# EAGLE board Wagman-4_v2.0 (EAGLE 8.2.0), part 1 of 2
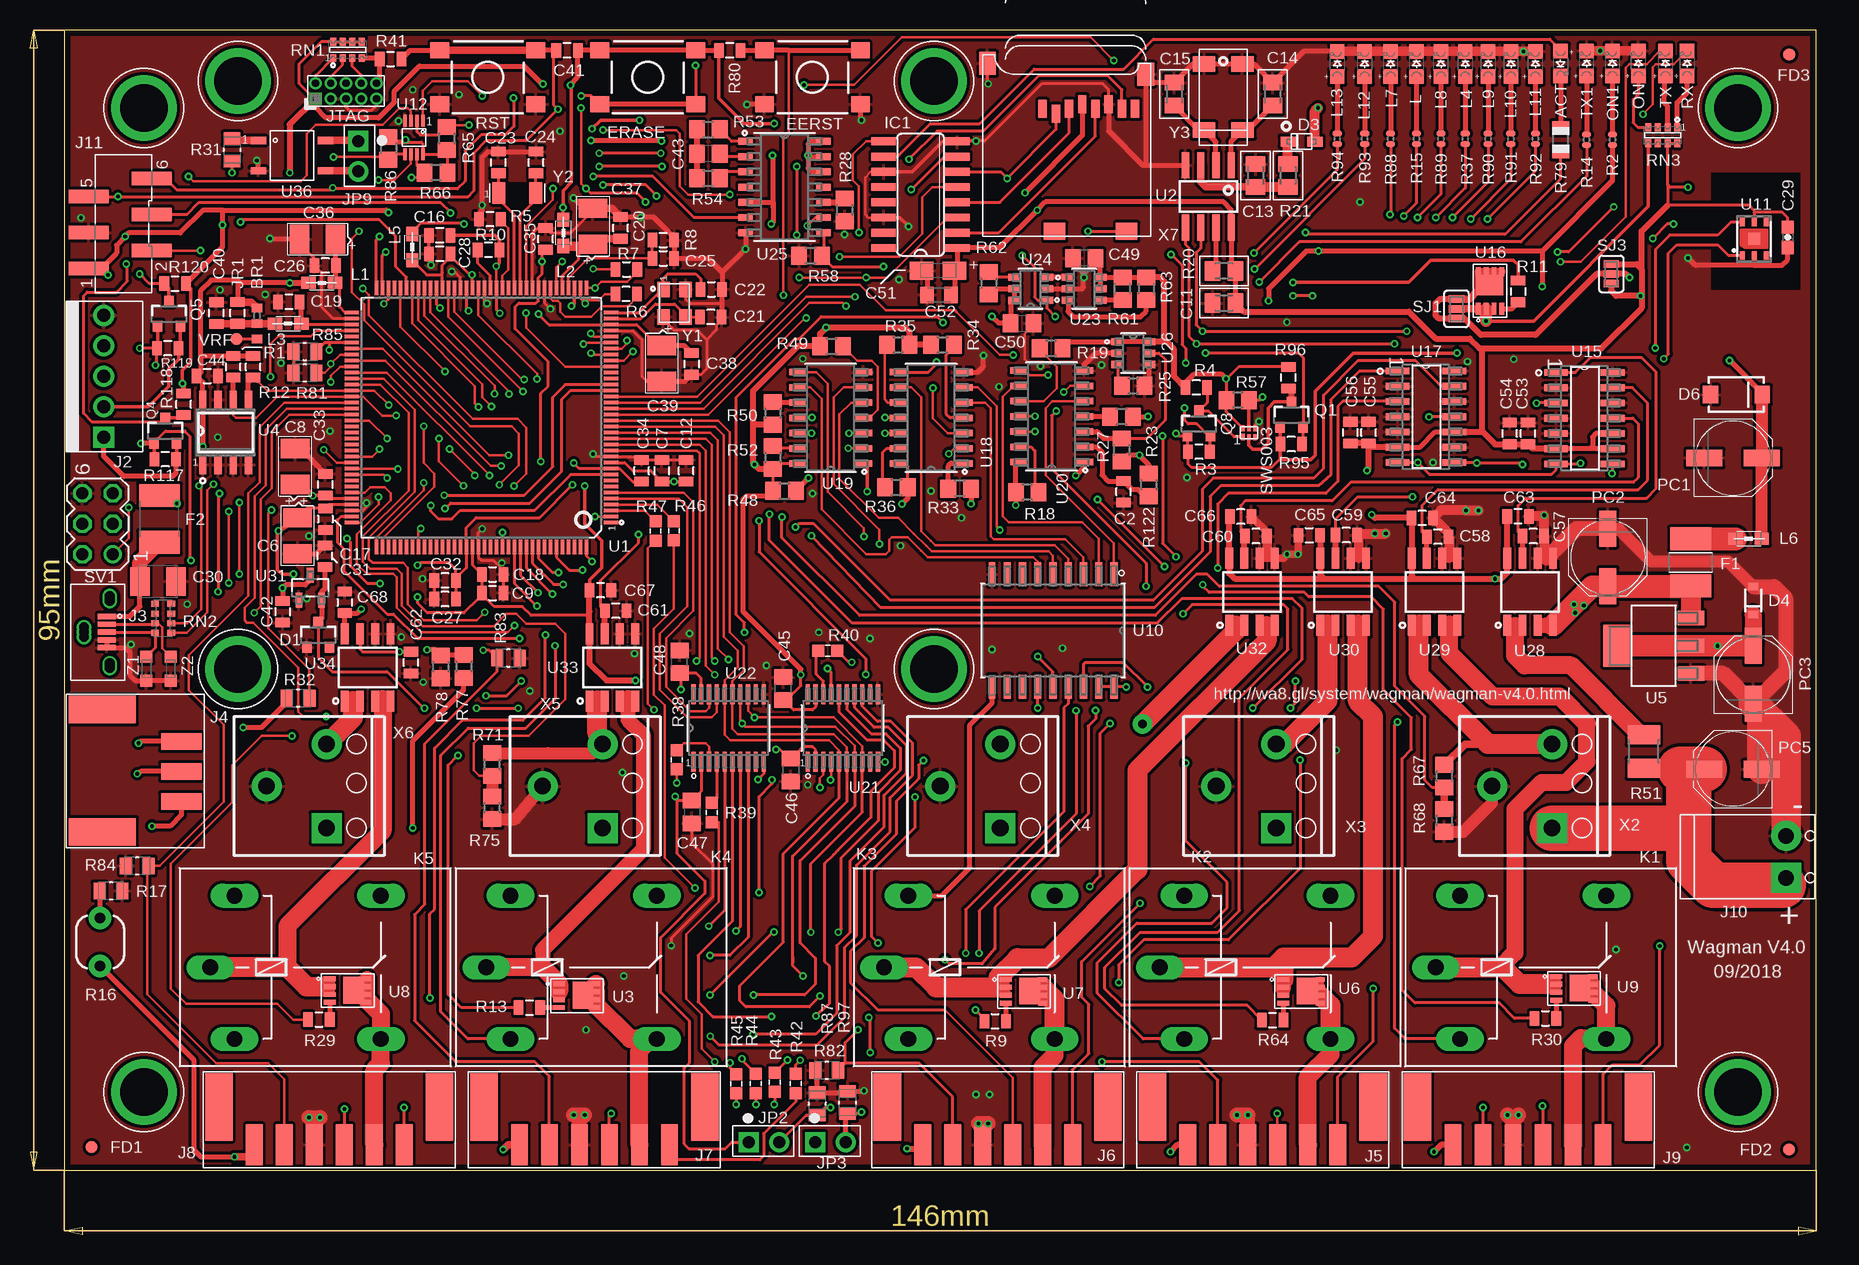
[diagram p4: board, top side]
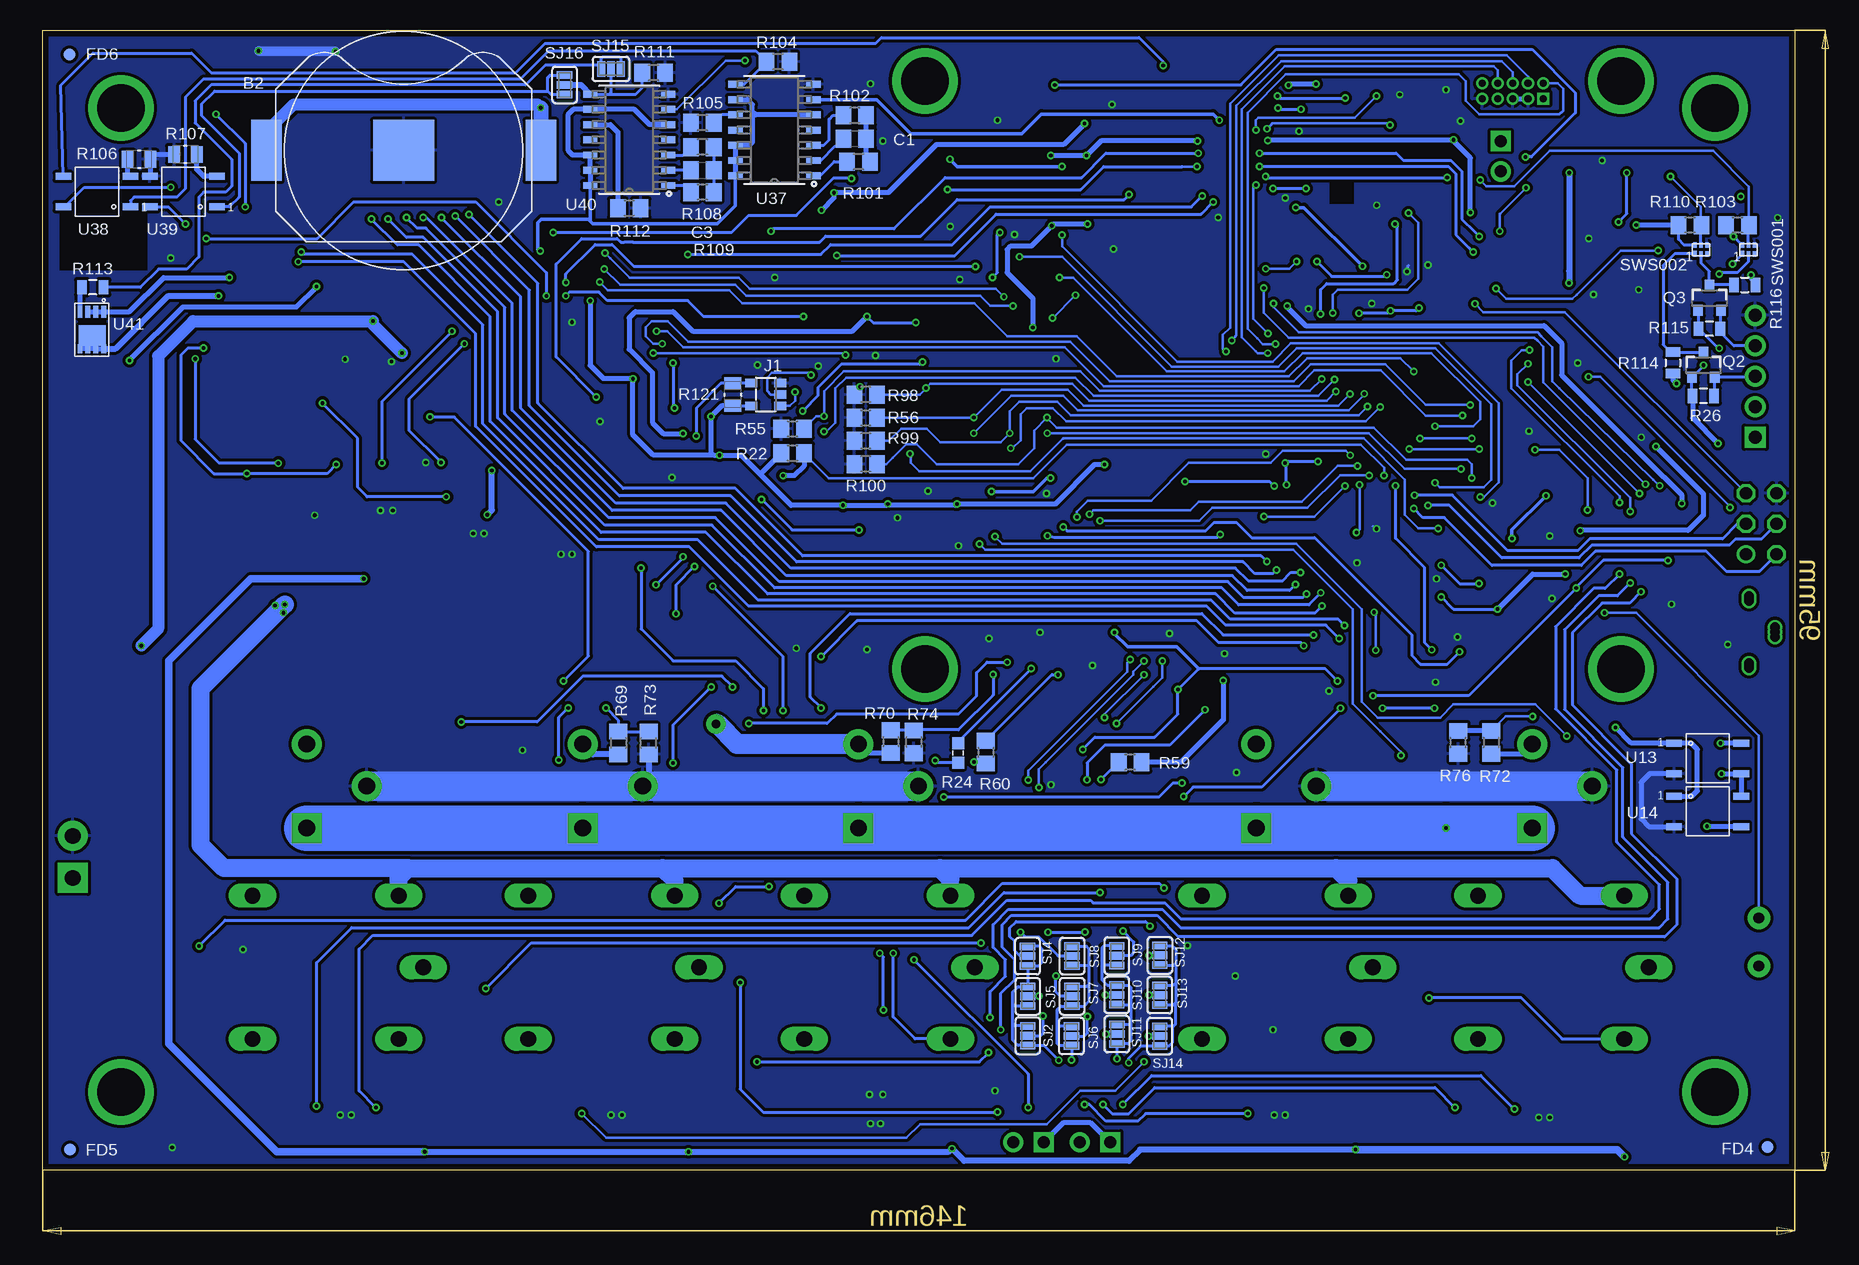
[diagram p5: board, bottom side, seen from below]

Size 148.84 x 100.38 mm. Coordinates in mm from the lower left corner, seen from the top.
Outline: 2.84,5.38 148.84,5.38 148.84,100.38 2.84,100.38 2.84,5.38
Copper layers (1*16): Top 0.035mm / dielectric 1.5mm / Bottom 0.035mm
Design rules "default *": minimum track width 0.2mm, minimum drill 12mil, track to track 10mil, track to pad 10mil, pad to pad 10mil, via to via 10mil, smd to smd 0mil, copper to edge 20mil, drill to drill 10mil, minimum pad ring 5mil, minimum via ring 5mil, stop-mask expansion 2.5mil, vias tented up to drill 0mil, thermal gap 10mil
tRestrict: area 140.1,78.7 to 147.5,88.5
bRestrict: area 140.1,80.4 to 147.4,85.3

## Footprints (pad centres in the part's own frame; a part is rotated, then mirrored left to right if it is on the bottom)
CHIPLED_0805 = smd 1.2 x 1.2: A 0,-1.05; C 0,1.05
BAT-HLD-002-SMT = smd 5.08 x 5.08: NEG 0,0 | smd 2.54 x 5.08: POS1 -11.43,0; POS2 11.43,0
J0402 = smd 0.7 x 0.9: 1 -0.65,0; 2 0.65,0; 3 1.95,0
C0805 = smd 1.3 x 1.5: 1 -0.95,0; 2 0.95,0
0805 = smd 0.8 x 1.2: 1 -0.9,0; 2 0.9,0
SMC_B = smd 1.6 x 2.4: + -1.5,0; - 1.5,0
M0805 = smd 1.3 x 1.6: 1 -0.95,0; 2 0.95,0
0603-CAP = smd 1.1 x 1: 1 -0.85,0; 2 0.85,0
A/3216-18R = smd 1.95 x 1.5: + 1.375,0; - -1.375,0
C0805K = smd 1.1 x 1.4: 1 -1,0; 2 1,0
SOT23-3 = smd 0.8 x 0.9: 1 -0.95,-1; 2 0.95,-1; 3 0,1.1
SOD-323F = smd 1.27 x 0.813: A -1.118,0; K 1.118,0
SOD-323 = smd 0.63 x 0.83: A 1.15,0; C -1.15,0
SMA-DIODE = smd 1.27 x 1.47: A -2.15,0; C 2.15,0
TACT_SPST_SMD_6X6 = smd 1.55 x 1.3: 1 -4,2.25; 2 4,2.25; 3 4,-2.25; 4 -4,-2.25
L1812 = smd 1.9 x 3.4: 1 -1.95,0; 2 1.95,0
FD-1MM = smd 1 x 1: 1 0,0
SO16 = smd 0.66 x 2.032: 1 -4.445,-3.073; 2 -3.175,-3.073; 3 -1.905,-3.073; 4 -0.635,-3.073; 5 0.635,-3.073; 6 1.905,-3.073; 7 3.175,-3.073; 8 4.445,-3.073; 9 4.445,3.073; 10 3.175,3.073; 11 1.905,3.073; 12 0.635,3.073; 13 -0.635,3.073; 14 -1.905,3.073; 15 -3.175,3.073; 16 -4.445,3.073
TSOP-5 = smd 0.7 x 1: 1 -0.95,-1.2; 2 0,-1.2; 3 0.95,-1.2; 4 0.95,1.2; 5 -0.95,1.2
01X05_P2.54_RELIMATE = drill 1.1 pad 1.778 square: 1 -5.08,0 | drill 1.1 pad 1.778: 2 -2.54,0; 3 0,0; 4 2.54,0; 5 5.08,0
1051330011_MINIUSB_VERTICAL = smd 0.45 x 1.5: 1 -1.3,0; 2 -0.65,0; 3 0,0; 4 0.65,0; 5 1.3,0 | drill 0.8: 6 -2.6,0.25; 7 3,0.25; 8 -3,0.25; 9 -2.8,0.25; 10 2.6,0.25; 11 2.8,0.25; 12 0.4,-1.9; 13 -0.4,-1.9; 14 0,-1.9
3PIN-PTSM-RA-2.5MM = smd 1.4 x 3.4: 1 -2.44,0; 2 0.06,0; 3 2.56,0 | smd 2.3 x 5.6: M1 -5.1,-6.6; M2 5.1,-6.6
6PIN-PTSM-2.5MM = smd 1.4 x 3.4: 1 -6.25,0; 2 -3.75,0; 3 -1.25,0; 4 1.25,0; 5 3.75,0; 6 6.25,0 | smd 2.3 x 5.6: M1 -9.2,-3.15; M2 9.2,-3.15
TB2-3.5MM = drill 1.3 pad 2.5 square: P$1 -1.75,0 | drill 1.3 pad 2.5: P$2 1.75,0
1X6-STRAIGHT-ALT = smd 1.1 x 3.3: 1 3.75,-2.9; 2 2.25,2.35; 3 0.75,-2.9; 4 -0.75,2.35; 5 -2.25,-2.9; 6 -3.75,2.35
CONN_2PIN_P2.54MM = drill 1 pad 1.676 square: 1 0,0 | drill 1 pad 1.676: 2 2.54,0
PINHEAD_2X05_127 = drill 0.6 pad 1.016 square: 1 -0.635,2.54 | drill 0.6 pad 1.016: 2 0.635,2.54; 3 -0.635,1.27; 4 0.635,1.27; 5 -0.635,0; 6 0.635,0; 7 -0.635,-1.27; 8 0.635,-1.27; 9 -0.635,-2.54; 10 0.635,-2.54
G5LE = drill 1.321 long: 1 -7.493,-5.969; 2 -7.493,5.969; O 4.699,5.969; P -9.525,0; S 4.699,-5.969
0805' = smd 1.2 x 1: 1 -1.1,0; 2 1.1,0
MH3.964 = drill 3.962 pad 5.461: 1 0,0
PANASONIC_D = smd 3 x 1.4: + 2.4,0; - -2.4,0
R0402 = smd 0.508 x 0.762: 1 -0.445,0; 2 0.445,0
PHOTOCELL-KIT = drill 0.9 pad 1.88: 1 -2,0; 2 2,0
RESC2013X65N = smd 1.016 x 1.397: 1 -0.94,0; 2 0.94,0
R0805 = smd 1.3 x 1.5: 1 -0.95,0; 2 0.95,0
PTC-0603 = smd 1 x 1: 1 -0.8,0; 2 0.8,0
R1210 = smd 1.6 x 2.7: 1 -1.4,0; 2 1.4,0
R0805' = smd 1.1 x 1.4: 1 -1,0; 2 1,0
CAT16 = smd 0.5 x 0.65: 1 -1.2,-0.675; 2 -0.4,-0.675; 3 0.4,-0.675; 4 1.2,-0.675; 5 1.2,0.675; 6 0.4,0.675; 7 -0.4,0.675; 8 -1.2,0.675
CAY16 = smd 0.5 x 0.65: 1 -1.2,-0.675; 2 -0.4,-0.675; 3 0.4,-0.675; 4 1.2,-0.675; 5 1.2,0.675; 6 0.4,0.675; 7 -0.4,0.675; 8 -1.2,0.675
SJ_3_PASTE1&2&3 = smd 0.635 x 1.27: 1 -0.813,0; 2 0,0; 3 0.813,0
MA03-2 = drill 1.016: 1 -2.54,-1.27 | drill 1.016 octagon: 2 -2.54,1.27; 3 0,-1.27; 4 0,1.27; 5 2.54,-1.27; 6 2.54,1.27
CAT872 = smd 0.3 x 0.53: 1 -0.5,-0.355 | smd 0.3 x 0.49: 2 0,-0.375; 3 0.5,-0.375; 4 0.5,0.375; 5 0,0.375; 6 -0.5,0.375
LQFP144 = smd 0.3 x 1.2: 1 -8.75,-10.8; 2 -8.25,-10.8; 3 -7.75,-10.8; 4 -7.25,-10.8; 5 -6.75,-10.8; 6 -6.25,-10.8; 7 -5.75,-10.8; 8 -5.25,-10.8; 9 -4.75,-10.8; 10 -4.25,-10.8; 11 -3.75,-10.8; 12 -3.25,-10.8; 13 -2.75,-10.8; 14 -2.25,-10.8; 15 -1.75,-10.8; 16 -1.25,-10.8; 17 -0.75,-10.8; 18 -0.25,-10.8; 19 0.25,-10.8; 20 0.75,-10.8; 21 1.25,-10.8; 22 1.75,-10.8; 23 2.25,-10.8; 24 2.75,-10.8; 25 3.25,-10.8; 26 3.75,-10.8; 27 4.25,-10.8; 28 4.75,-10.8; 29 5.25,-10.8; 30 5.75,-10.8; 31 6.25,-10.8; 32 6.75,-10.8; 33 7.25,-10.8; 34 7.75,-10.8; 35 8.25,-10.8; 36 8.75,-10.8; 73 8.75,10.8; 74 8.25,10.8; 75 7.75,10.8; 76 7.25,10.8; 77 6.75,10.8; 78 6.25,10.8; 79 5.75,10.8; 80 5.25,10.8; 81 4.75,10.8; 82 4.25,10.8; 83 3.75,10.8; 84 3.25,10.8; 85 2.75,10.8; 86 2.25,10.8; 87 1.75,10.8; 88 1.25,10.8; 89 0.75,10.8; 90 0.25,10.8; 91 -0.25,10.8; 92 -0.75,10.8; 93 -1.25,10.8; 94 -1.75,10.8; 95 -2.25,10.8; 96 -2.75,10.8; 97 -3.25,10.8; 98 -3.75,10.8; 99 -4.25,10.8; 100 -4.75,10.8; 101 -5.25,10.8; 102 -5.75,10.8; 103 -6.25,10.8; 104 -6.75,10.8; 105 -7.25,10.8; 106 -7.75,10.8; 107 -8.25,10.8; 108 -8.75,10.8 | smd 1.2 x 0.3: 37 10.8,-8.75; 38 10.8,-8.25; 39 10.8,-7.75; 40 10.8,-7.25; 41 10.8,-6.75; 42 10.8,-6.25; 43 10.8,-5.75; 44 10.8,-5.25; 45 10.8,-4.75; 46 10.8,-4.25; 47 10.8,-3.75; 48 10.8,-3.25; 49 10.8,-2.75; 50 10.8,-2.25; 51 10.8,-1.75; 52 10.8,-1.25; 53 10.8,-0.75; 54 10.8,-0.25; 55 10.8,0.25; 56 10.8,0.75; 57 10.8,1.25; 58 10.8,1.75; 59 10.8,2.25; 60 10.8,2.75; 61 10.8,3.25; 62 10.8,3.75; 63 10.8,4.25; 64 10.8,4.75; 65 10.8,5.25; 66 10.8,5.75; 67 10.8,6.25; 68 10.8,6.75; 69 10.8,7.25; 70 10.8,7.75; 71 10.8,8.25; 72 10.8,8.75; 109 -10.8,8.75; 110 -10.8,8.25; 111 -10.8,7.75; 112 -10.8,7.25; 113 -10.8,6.75; 114 -10.8,6.25; 115 -10.8,5.75; 116 -10.8,5.25; 117 -10.8,4.75; 118 -10.8,4.25; 119 -10.8,3.75; 120 -10.8,3.25; 121 -10.8,2.75; 122 -10.8,2.25; 123 -10.8,1.75; 124 -10.8,1.25; 125 -10.8,0.75; 126 -10.8,0.25; 127 -10.8,-0.25; 128 -10.8,-0.75; 129 -10.8,-1.25; 130 -10.8,-1.75; 131 -10.8,-2.25; 132 -10.8,-2.75; 133 -10.8,-3.25; 134 -10.8,-3.75; 135 -10.8,-4.25; 136 -10.8,-4.75; 137 -10.8,-5.25; 138 -10.8,-5.75; 139 -10.8,-6.25; 140 -10.8,-6.75; 141 -10.8,-7.25; 142 -10.8,-7.75; 143 -10.8,-8.25; 144 -10.8,-8.75
SO08 = smd 0.6 x 2.2: 1 -1.905,-2.6; 2 -0.635,-2.6; 3 0.635,-2.6; 4 1.905,-2.6; 5 1.905,2.6; 6 0.635,2.6; 7 -0.635,2.6; 8 -1.905,2.6
SIS413 = smd 0.99 x 0.405: 1 0,0; 2 0,-0.66; 3 0,-1.32; 4 0,-1.98 | smd 0.76 x 0.405: 5 3.075,-1.98; 6 3.075,-1.32; 7 3.075,-0.66; 8 3.075,0 | smd 1.725 x 2.235: PAD 1.992,-0.96
SOIC8 = smd 0.6 x 1.55: 1 -1.905,-2.7; 2 -0.635,-2.7; 3 0.635,-2.7; 4 1.905,-2.7; 5 1.905,2.7; 6 0.635,2.7; 7 -0.635,2.7; 8 -1.905,2.7
SOT230P700X180-4N = smd 2.2 x 1.2: 1 -3.1,2.311; 2 -3.1,0; 3 -3.1,-2.311 | smd 2.2 x 3.5: 4 3.1,0
DW18 = smd 2 x 0.6: 1 -4.7,5.08; 2 -4.7,3.81; 3 -4.7,2.54; 4 -4.7,1.27; 5 -4.7,0; 6 -4.7,-1.27; 7 -4.7,-2.54; 8 -4.7,-3.81; 11 4.7,-3.81; 12 4.7,-2.54; 13 4.7,-1.27; 14 4.7,0; 15 4.7,1.27; 16 4.7,2.54; 17 4.7,3.81; 18 4.7,5.08 | smd 1.95 x 0.55: 9 -4.7,-5.08; 10 4.7,-5.08
DD8-3X3MM = smd 0.4 x 0.7: 1 -1,-1.4; 2 0,-1.4; 3 1,-1.4; 4 1,1.4; 5 0,1.4; 6 -1,1.4 | smd 1 x 1: EXP 0,0
US-8 = smd 0.3 x 1: 1 -0.75,-1.4; 2 -0.25,-1.4; 3 0.25,-1.4; 4 0.75,-1.4; 5 0.75,1.4; 6 0.25,1.4; 7 -0.25,1.4; 8 -0.75,1.4
SOP-4 = smd 1.3 x 0.6: 1 0,0; 2 0,-2.54; 3 5.6,-2.54; 4 5.6,0
SOIC127P600X175-14N = smd 1.981 x 0.559: 1 -2.362,3.81; 2 -2.362,2.54; 3 -2.362,1.27; 4 -2.362,0; 5 -2.362,-1.27; 6 -2.362,-2.54; 7 -2.362,-3.81; 8 2.362,-3.81; 9 2.362,-2.54; 10 2.362,-1.27; 11 2.362,0; 12 2.362,1.27; 13 2.362,2.54; 14 2.362,3.81
D14 = smd 1.5 x 0.55: 1 -2.7,3.81; 2 -2.7,2.54; 3 -2.7,1.27; 4 -2.7,0; 5 -2.7,-1.27; 6 -2.7,-2.54; 7 -2.7,-3.81; 8 2.7,-3.81; 9 2.7,-2.54; 10 2.7,-1.27; 11 2.7,0; 12 2.7,1.27; 13 2.7,2.54; 14 2.7,3.81
PW20 = smd 1.676 x 0.356: 1 -2.819,2.925; 2 -2.819,2.275; 3 -2.819,1.625; 4 -2.819,0.975; 5 -2.819,0.325; 6 -2.819,-0.325; 7 -2.819,-0.975; 8 -2.819,-1.625; 9 -2.819,-2.275; 10 -2.819,-2.925; 11 2.819,-2.925; 12 2.819,-2.275; 13 2.819,-1.625; 14 2.819,-0.975; 15 2.819,-0.325; 16 2.819,0.325; 17 2.819,0.975; 18 2.819,1.625; 19 2.819,2.275; 20 2.819,2.925
DBV6 = smd 1.05 x 0.6: 1 -1.35,0.95; 2 -1.35,0; 3 -1.35,-0.95; 4 1.35,-0.95; 5 1.35,0; 6 1.35,0.95
SOIC14-3.9MM = smd 1.2 x 0.58: 1 -3.25,3.81; 2 -3.25,2.54; 3 -3.25,1.27; 4 -3.25,0; 5 -3.25,-1.27; 6 -3.25,-2.54; 7 -3.25,-3.81; 8 3.25,-3.81; 9 3.25,-2.54; 10 3.25,-1.27; 11 3.25,0; 12 3.25,1.27; 13 3.25,2.54; 14 3.25,3.81
DDC6 = smd 1.05 x 0.6: 1 -1.3,0.95; 2 -1.3,0; 3 -1.3,-0.95; 4 1.3,-0.95; 5 1.3,0; 6 1.3,0.95
SOIC-8 = smd 1.75 x 0.65: 1 -2.8,1.905; 2 -2.8,0.635; 3 -2.8,-0.635; 4 -2.8,-1.905; 5 2.8,-1.905; 6 2.8,-0.635; 7 2.8,0.635; 8 2.8,1.905
SOT95P237X112-3N = smd 0.559 x 1.27: 1 -0.94,-1.041; 2 0.94,-1.041; 3 0,1.041
1-2834019-3 = drill 1.4 pad 2.5 square: 1 -3.5,0 | drill 1.4 pad 2.5: 2 0,5; 3 3.5,0
MICROSD = smd 0.7 x 1.5: 1 9,-10.64; 2 7.9,-10.24; 3 6.8,-10.64; 4 5.7,-11.04; 5 4.6,-10.64; 6 3.5,-11.04; 7 2.4,-10.64; 8 1.3,-10.64 | smd 1.8 x 1.4: CD1 2,-0.44; CD2 8,-0.44 | smd 1.4 x 1.9: MT1 0.4,-13.54; MT2 13.6,-14.44
CRYSTAL-3.2-2.5 = smd 1.3 x 1.05: 1 -1.15,-0.925; 2 1.15,-0.925; 3 1.15,0.925; 4 -1.15,0.925
RESONATOR_EPSON_FC_145 = smd 1.1 x 1.8: P$1 -1.55,0; P$2 1.55,0
CRYSTAL-CITIZEN-CM2XXC = smd 1.3 x 1.9: P$1 -2.75,-1.6; P$2 2.75,-1.6; P$3 2.75,1.6; P$4 -2.75,1.6
CT/CN0603 = smd 1 x 1: 1 -1,0; 2 1,0

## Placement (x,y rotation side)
ACT  RED  [CHIPLED_0805]  127.55,97.58 180 top
B2  CR2016  [BAT-HLD-002-SMT]  118.77,90.34 180 bottom
BR1  NM  [J0402]  18.92,75.27 90 top
C1  10nF  [C0805]  81.17,91.33 0 bottom
C2  10uF  [0805]  91.13,61.89 90 top
C3  10nF  [C0805]  93.87,88.69 0 bottom
C6  10u  [SMC_B]  22.29,58.24 270 top
C7  100nF  [0805]  52.65,63.65 90 top
C8  10u  [SMC_B]  22.09,64.01 90 top
C9  100nF  [0805]  38.55,53.46 0 top
C11  100nF  [M0805]  99.49,77.62 180 top
C12  100nF  [0805]  54.68,63.65 90 top
C13  100pF  [M0805]  102.13,88.26 90 top
C14  10pF  [M0805]  103.55,95.04 90 top
C15  8.2pF  [M0805]  95.35,95.04 90 top
C16  100nF  [0805]  34.15,83.26 180 top
C17  100nF  [0805]  24.61,59.62 270 top
C18  100nF  [0805]  38.55,55.01 0 top
C19  100nF  [0805]  21.57,77.72 180 top
C20  100nF  [0805]  49.22,83.88 90 top
C21  22pF  [0805]  56.74,76.46 180 top
C22  22pF  [0805]  56.78,78.76 0 top
C23  22pF  [0805]  39.03,89.35 90 top
C24  22pF  [0805]  42.18,89.35 90 top
C25  22pF  [0805]  52.77,81.35 0 top
C26  100nF  [0805]  24.6,80.75 180 top
C27  100nF  [0805]  34.59,52.96 180 top
C28  100nF  [0805]  34.14,81.73 180 top
C29  100nF  [0603-CAP]  146.48,83.1 270 top
C30  10nF  [SMC_B]  10.66,54.43 0 top
C31  1uF  [0805]  24.57,56.54 90 top
C32  100nF  [0805]  34.59,54.51 180 top
C33  100nF  [0805]  24.61,62.5 90 top
C34  100nF  [0805]  50.97,63.65 90 top
C35  100nF  [0805]  42.97,82.97 90 top
C36  10u  [SMC_B]  23.96,82.94 180 top
C37  10u  [SMC_B]  46.91,84.03 90 top
C38  100nF  [0805]  55.13,72.55 270 top
C39  10u  [SMC_B]  52.64,72.59 270 top
C40  100nF  [0805]  15.53,76.79 90 top
C41  10nF  [0805]  44.75,98.69 180 top
C42  1uF  [0805]  21.05,51.9 270 top
C43  10nF  [C0805]  56.53,90.06 180 top
C44  100nF  [0805]  14.78,71.55 0 top
C45  0.1uF  [C0805]  62.78,45.51 90 top
C46  0.1uF  [C0805]  63.39,38.71 270 top
C47  0.1uF  [C0805]  55.16,35.22 270 top
C48  0.1uF  [C0805]  54.13,47.73 90 top
C49  0.1uF  [C0805]  87.86,81.35 180 top
C50  0.1uF  [C0805]  82.66,75.95 0 top
C51  10uF/10V  [A/3216-18R]  75.68,80.33 0 top
C52  0.1uF  [C0805K]  75.76,78.3 180 top
C53  0.1uF  [0805]  124.84,66.76 90 top
C54  10uF  [0805]  123.31,66.76 90 top
C55  0.1uF  [0805]  111.55,66.83 90 top
C56  10uF  [0805]  110.03,66.83 90 top
C57  1nF  [0805]  125.27,58.2 180 top
C58  1nF  [0805]  117.31,58.15 180 top
C59  1nF  [0805]  109.69,58.28 180 top
C60  1nF  [0805]  102.16,58.2 180 top
C61  1nF  [0805]  48.81,51.98 180 top
C62  1nF  [0805]  31.75,47.66 90 top
C63  0.1uF  [0805]  124,59.86 180 top
C64  0.1uF  [0805]  116.03,59.72 180 top
C65  0.1uF  [0805]  106.61,58.27 0 top
C66  0.1uF  [0805]  100.89,59.83 180 top
C67  0.1uF  [0805]  47.54,53.69 180 top
C68  0.1uF  [0805]  26.23,52.68 270 top
D1  BZX84C2V4LT1GOSCT-ND  [SOT23-3]  24.02,49.95 0 top
D3  PMEG6002EJ  [SOD-323F]  105.96,91.08 180 top
D4  MM3Z3V6T1GOSCT-ND  [SOD-323]  143.6,52.84 90 top
D6  SMAZ5V6-FDICT-ND  [SMA-DIODE]  142.2,70 0 top
DRILEGEND  [DRILEGEND]  not placed on the board
EERST  PTS65SM43SMTR92LFS  [TACT_SPST_SMD_6X6]  65.2,96.44 0 top
ERASE  PTS65SM43SMTR92LFS  [TACT_SPST_SMD_6X6]  51.48,96.44 0 top
F1  MF-MSMF050-2 500mA  [L1812]  138.39,56.03 270 top
F2  MF-MSMF050-2 500mA  [L1812]  10.79,59.63 90 top
FD1  FIDUCIAL-1MM  [FD-1MM]  5.13,7.29 0 top
FD2  FIDUCIAL-1MM  [FD-1MM]  146.58,7.08 0 top
FD3  FIDUCIAL-1MM  [FD-1MM]  146.6,98.34 0 top
FD4  FIDUCIAL-1MM  [FD-1MM]  5.13,7.29 0 bottom
FD5  FIDUCIAL-1MM  [FD-1MM]  146.58,7.08 0 bottom
FD6  FIDUCIAL-1MM  [FD-1MM]  146.6,98.34 0 bottom
IC1  4050D  [SO16]  74.21,86.66 90 top
J1  MC74VHC1G09DTT1G  [TSOP-5]  88.59,70 90 bottom
J2  022232051  [01X05_P2.54_RELIMATE]  6.14,71.52 90 top
J3  1051330011_MINIUSB  [1051330011_MINIUSB_VERTICAL]  6.4,50.21 270 top
J4  PXC_277-2066-1-ND  [3PIN-PTSM-RA-2.5MM]  12.62,38.65 270 top
J5  PXC-277-2076-1-ND  [6PIN-PTSM-2.5MM]  102.74,7.48 180 top
J6  PXC-277-2076-1-ND  [6PIN-PTSM-2.5MM]  80.64,7.48 180 top
J7  PXC-277-2076-1-ND  [6PIN-PTSM-2.5MM]  47.04,7.48 180 top
J8  PXC-277-2076-1-ND  [6PIN-PTSM-2.5MM]  24.94,7.48 180 top
J9  PXC-277-2076-1-ND  [6PIN-PTSM-2.5MM]  124.84,7.48 180 top
J10  277-1779-ND  [TB2-3.5MM]  146.34,31.48 90 top
J11  292231-6  [1X6-STRAIGHT-ALT]  7.79,84.25 270 top
JP2  [CONN_2PIN_P2.54MM]  59.89,7.69 0 top
JP3  [CONN_2PIN_P2.54MM]  65.43,7.69 0 top
JP9  [CONN_2PIN_P2.54MM]  27.34,91.13 270 top
JR1  0R  [0805]  17.29,76.8 90 top
JTAG  [PINHEAD_2X05_127]  26.34,95.3 90 top
K1  G5LE  [G5LE]  126.67,22.27 0 top
K2  G5LE  [G5LE]  103.68,22.27 0 top
K3  G5LE  [G5LE]  80.69,22.27 0 top
K4  G5LE  [G5LE]  47.54,22.27 0 top
K5  G5LE  [G5LE]  24.54,22.27 0 top
L  green  [CHIPLED_0805]  115.54,97.54 0 top
L1  MH2029-300Y  [0805']  24.32,79.3 0 top
L2  MH2029-300Y  [0805']  44.45,83.47 270 top
L3  MH2029-300Y  [0805']  21.51,75.92 0 top
L4  green  [CHIPLED_0805]  119.61,97.54 0 top
L5  MH2029-300Y  [0805']  31.85,82.29 90 top
L6  MH2029-300Y  [0805']  143.21,57.98 180 top
L7  green  [CHIPLED_0805]  113.38,97.54 0 top
L8  green  [CHIPLED_0805]  117.57,97.54 0 top
L9  green  [CHIPLED_0805]  121.51,97.54 0 top
L10  green  [CHIPLED_0805]  123.42,97.54 0 top
L11  green  [CHIPLED_0805]  125.45,97.54 0 top
L12  green  [CHIPLED_0805]  111.22,97.54 0 top
L13  green  [CHIPLED_0805]  108.94,97.54 0 top
MH1  MH-3.964  [MH3.964]  9.48,11.89 0 top
MH2  MH-3.964  [MH3.964]  9.48,93.88 0 top
MH3  MH-3.964  [MH3.964]  142.34,93.88 0 top
MH4  MH-3.964  [MH3.964]  142.34,11.89 0 top
MH5  MH-3.964  [MH3.964]  17.34,96.13 0 top
MH6  MH-3.964  [MH3.964]  75.34,96.13 0 top
MH7  MH-3.964  [MH3.964]  75.34,47.13 0 top
MH8  MH-3.964  [MH3.964]  17.34,47.13 0 top
ON  GREEN  [CHIPLED_0805]  134.03,97.58 0 top
ON1  blue  [CHIPLED_0805]  131.87,97.58 0 top
PC1  47u  [PANASONIC_D]  141.92,64.71 0 top
PC2  4.7uF  [PANASONIC_D]  131.49,56.43 270 top
PC3  1uF  [PANASONIC_D]  143.6,46.66 90 top
PC5  47u  [PANASONIC_D]  141.91,38.78 180 top
Q1  BSS138  [SOT23-3]  105.12,68.28 0 top
Q2  BSS138  [SOT23-3]  10.46,72.44 0 bottom
Q3  BSS138  [SOT23-3]  9.95,78.02 0 bottom
Q4  BSS138  [SOT23-3]  11.27,66.95 0 top
Q5  BSS138  [SOT23-3]  11.58,76.7 0 top
Q8  BSS138  [SOT23-3]  97.41,67.55 0 top
R1  4.7K  [0805]  16.94,72.31 90 top
R2  1K  [R0402]  131.87,91.23 90 top
R3  10K  [0805]  97.41,65.24 180 top
R4  4.7K  [0805]  97.19,70.59 180 top
R5  0R_NM  [0805]  38.33,84.61 180 top
R6  39R 1%  [0805]  49.68,78.38 180 top
R7  39R 1%  [0805]  49.7,80.43 0 top
R8  6K8 1%  [0805]  52.77,82.88 0 top
R9  1k  [0805]  80.43,17.77 0 top
R10  100k  [0805]  38.21,82.05 180 top
R11  1k  [0805]  124.01,78.59 270 top
R12  4.7K  [0805]  18.59,72.31 90 top
R13  1k  [0805]  41.62,18.92 0 top
R14  1K  [R0402]  129.71,91.23 90 top
R15  1K  [R0402]  115.54,91.32 90 top
R16  PHOTOCELLPTH-KIT  [PHOTOCELL-KIT]  5.84,24.38 90 top
R17  23K  [RESC2013X65N]  6.75,28.64 0 top
R18  10K  [R0805]  83.11,61.86 180 top
R19  10K  [R0805]  85.1,73.87 0 top
R20  10K  [M0805]  99.49,80.29 0 top
R21  1K  [M0805]  104.83,88.25 90 top
R22  10K  [R0805]  86.36,65.12 0 bottom
R23  10K  [R0805]  90.95,68.16 180 top
R24  PRG18BB470MB1RB  [PTC-0603]  72.56,40.13 90 bottom
R25  22.021K  [R0805]  91.94,70.74 0 top
R26  10K  [0805]  10.46,69.9 180 bottom
R27  10K  [R0805]  90.96,65.37 270 top
R28  10K  [R0805]  67.88,85.39 270 top
R29  1k  [0805]  24.08,17.92 0 top
R30  1K  [0805]  126.28,18.02 0 top
R31  150R  [RESC2013X65N]  16.84,90.39 270 top
R32  150R  [RESC2013X65N]  22.35,44.7 0 top
R33  10K  [R0805]  77.47,62.17 180 top
R34  10K  [R0805]  76.04,74.16 0 top
R35  10K  [R0805]  72.36,74.16 0 top
R36  10K  [R0805]  72.2,62.27 0 top
R37  1K  [R0402]  119.61,91.32 90 top
R38  PRG18BB470MB1RB  [PTC-0603]  53.91,39.58 90 top
R39  PRG18BB470MB1RB  [PTC-0603]  56.81,35.17 90 top
R40  PRG18BB470MB1RB  [PTC-0603]  66.49,48.66 180 top
R41  0R  [0805]  30.04,97.96 0 top
R42  PRG18BB470MB1RB  [PTC-0603]  63.81,12.59 90 top
R43  PRG18BB470MB1RB  [PTC-0603]  62.07,12.7 90 top
R44  PRG18BB470MB1RB  [PTC-0603]  60.49,12.6 90 top
R45  PRG18BB470MB1RB  [PTC-0603]  58.85,12.57 90 top
R46  PRG18BB470MB1RB  [PTC-0603]  53.67,58.66 90 top
R47  PRG18BB470MB1RB  [PTC-0603]  52.13,58.63 90 top
R48  10K  [R0805]  62.87,61.97 0 top
R49  10K  [R0805]  66.79,74.03 0 top
R50  10K  [R0805]  61.89,68.44 270 top
R51  BLE32P  [R1210]  134.49,40.25 90 top
R52  10K  [R0805]  61.89,64.75 270 top
R53  20K  [R0805]  56.53,92.09 0 top
R54  40.2K  [R0805]  56.53,88.03 0 top
R55  10K  [R0805]  86.36,67.15 0 bottom
R56  10K  [R0805]  80.26,68.07 0 bottom
R57  20K  [R0805]  100.65,69.54 180 top
R58  10K  [R0805]  65.03,81.58 0 top
R59  100K  [R0805]  58.23,39.37 180 bottom
R60  100K  [R0805]  70.26,40.2 270 bottom
R61  100K  [R0805]  91.04,78.81 90 top
R62  100K  [R0805]  79.9,79.28 270 top
R63  10K  [R0805]  93.01,78.81 270 top
R64  1k  [0805]  103.55,17.87 0 top
R65  10K  [R0805]  34.74,91.33 90 top
R66  10K  [R0805]  33.83,88.49 180 top
R67  17K  [R0805]  117.87,38.2 90 top
R68  3K  [R0805]  117.87,34.52 90 top
R69  17K  [R0805]  100.87,40.97 270 bottom
R70  17K  [R0805]  78.18,41.07 270 bottom
R71  17K  [R0805]  38.52,39.18 90 top
R72  17K  [R0805]  28.14,41.02 270 bottom
R73  3K  [R0805]  98.36,40.96 90 bottom
R74  3K  [R0805]  76.24,41.06 90 bottom
R75  3K  [R0805]  38.52,35.57 90 top
R76  3K  [R0805]  30.88,41.02 90 bottom
R77  17K  [R0805]  36.14,47.33 270 top
R78  3K  [R0805]  34.25,47.31 90 top
R79  1K  [R0805']  127.55,91.23 90 top
R80  1k  [0805]  58.31,98.69 180 top
R81  23K  [RESC2013X65N]  22.91,71.8 180 top
R82  23K  [RESC2013X65N]  66.4,13.68 180 top
R83  23K  [RESC2013X65N]  39.87,48.05 0 top
R84  23K  [RESC2013X65N]  8.94,30.72 180 top
R85  23K  [RESC2013X65N]  22.91,73.58 180 top
R86  10K  [R0805]  29.87,90.52 270 top
R87  150R  [RESC2013X65N]  65.61,10.89 270 top
R88  1K  [R0402]  113.38,91.32 90 top
R89  1K  [R0402]  117.57,91.32 90 top
R90  1K  [R0402]  121.51,91.32 90 top
R91  1K  [R0402]  123.4,91.32 90 top
R92  1K  [R0402]  125.45,91.32 90 top
R93  1K  [R0402]  111.22,91.32 90 top
R94  1K  [R0402]  108.94,91.32 90 top
R95  10K  [0805]  105.1,65.87 180 top
R96  4.7K  [0805]  104.87,71.41 90 top
R97  150R  [RESC2013X65N]  68.13,11 270 top
R98  10K  [R0805]  80.26,70 180 bottom
R99  10K  [R0805]  80.26,66.14 180 bottom
R100  10K  [R0805]  80.26,64.21 180 bottom
R101  20K  [R0805]  80.87,89.4 180 bottom
R102  40.2K  [R0805]  81.17,93.26 180 bottom
R103  20K  [R0805]  7.62,84.12 180 bottom
R104  10K  [R0805]  87.57,97.73 180 bottom
R105  10K  [R0805]  93.87,92.65 180 bottom
R106  150R  [RESC2013X65N]  140.81,89.61 0 bottom
R107  150R  [RESC2013X65N]  136.95,90.01 180 bottom
R108  20K  [R0805]  93.87,86.86 180 bottom
R109  40.2K  [R0805]  93.87,90.62 180 bottom
R110  20K  [R0805]  11.58,84.12 180 bottom
R111  10K  [R0805]  97.94,96.82 180 bottom
R112  10K  [R0805]  99.97,85.54 0 bottom
R113  1k  [0805]  144.67,78.94 180 bottom
R114  4.7K  [0805]  13,72.64 270 bottom
R115  10K  [0805]  9.95,75.48 180 bottom
R116  4.7K  [0805]  7.01,79.14 0 bottom
R117  10K  [0805]  11.27,64.61 180 top
R118  4.7K  [0805]  12.8,69.18 90 top
R119  10K  [0805]  11.48,73.86 180 top
R120  4.7K  [0805]  12.09,79.24 0 top
R121  10K  [RESC2013X65N]  91.33,70 270 bottom
R122  1M  [R0805]  93.24,62.48 90 top
RN1  100K  [CAT16]  26.46,98.72 0 top
RN2  22R  [CAY16]  11.1,51.35 90 top
RN3  1k  [CAT16]  136.06,91.61 180 top
RST  PTS65SM43SMTR92LFS  [TACT_SPST_SMD_6X6]  38.15,96.44 0 top
RX  YELLOW  [CHIPLED_0805]  138.09,97.58 0 top
SJ1  [SJ_3_PASTE1&2&3]  118.88,77.14 90 top
SJ2  [SJ_3_PASTE1&2&3]  66.76,16.57 270 bottom
SJ3  [SJ_3_PASTE1&2&3]  131.77,80.06 270 top
SJ4  [SJ_3_PASTE1&2&3]  66.78,23.2 90 bottom
SJ5  [SJ_3_PASTE1&2&3]  66.76,19.86 270 bottom
SJ6  [SJ_3_PASTE1&2&3]  63.11,16.54 90 bottom
SJ7  [SJ_3_PASTE1&2&3]  63.07,19.86 270 bottom
SJ8  [SJ_3_PASTE1&2&3]  63.07,23.22 270 bottom
SJ9  [SJ_3_PASTE1&2&3]  59.35,23.24 270 bottom
SJ10  [SJ_3_PASTE1&2&3]  59.34,19.97 90 bottom
SJ11  [SJ_3_PASTE1&2&3]  59.33,16.7 90 bottom
SJ12  [SJ_3_PASTE1&2&3]  55.75,23.27 270 bottom
SJ13  [SJ_3_PASTE1&2&3]  55.76,19.95 90 bottom
SJ14  [SJ_3_PASTE1&2&3]  55.77,16.54 270 bottom
SJ15  [SJ_3_PASTE1&2&3]  101.49,97.12 180 bottom
SJ16  [SJ_3_PASTE1&2&3]  105.35,95.8 270 bottom
SV1  [MA03-2]  5.63,59.23 90 top
SWS001  CAT872  [CAT872]  6.7,82.09 0 bottom
SWS002  CAT872  [CAT872]  10.66,82.09 0 bottom
SWS003  CAT872  [CAT872]  101.57,66.82 0 top
TX  YELLOW  [CHIPLED_0805]  136.29,97.58 0 top
TX1  yellow  [CHIPLED_0805]  129.71,97.58 0 top
U1  ATSAM3X8EA-AU  [LQFP144]  37.61,68.09 90 top
U2  MCP79412  [SO08]  98.2,86.51 180 top
U3  SIS413DN  [SIS413]  44.09,20.9 0 top
U4  24LC256T-E/SN  [SOIC8]  16.3,66.85 0 top
U5  AZ1117EH-3.3TRG1  [SOT230P700X180-4N]  135.3,49.07 180 top
U6  SIS413DN  [SIS413]  104.44,21.25 0 top
U7  SIS413DN  [SIS413]  81.33,21.25 0 top
U8  SIS413DN  [SIS413]  24.99,21.32 0 top
U9  SIS413DN  [SIS413]  127.17,21.51 0 top
U10  ULN2803ADWR  [DW18]  85.25,50.34 270 top
U11  HTU21D  [DD8-3X3MM]  143.68,82.98 0 top
U12  NL37WZ06USG  [US-8]  32,91.44 180 top
U13  CPC1125N  [SOP-4]  12.9,40.95 0 bottom
U14  CPC1017N  [SOP-4]  12.9,36.53 0 bottom
U15  MCP3428-E/SL  [SOIC127P600X175-14N]  129.53,68.03 0 top
U16  SIS413DN  [SIS413]  120.68,77.15 90 top
U17  MCP3428-E/SL  [SOIC127P600X175-14N]  116.33,68.16 0 top
U18  SN74HCT74DR  [D14]  75.1,68.06 180 top
U19  SN74HCT74DR  [D14]  66.72,68.06 180 top
U20  SN74HCT74DR  [D14]  85.13,68.18 180 top
U21  TXS0108EPWR  [PW20]  67.74,42.21 90 top
U22  TXS0108EPWR  [PW20]  58.21,42.21 90 top
U23  TPS3808G50DBVR  [DBV6]  87.86,78.81 0 top
U24  TPS3808G50DBVR  [DBV6]  83.38,78.81 180 top
U25  MC14541BDR2G  [SOIC14-3.9MM]  62.88,87.3 0 top
U26  TPL5110QDDCRQ1  [DDC6]  91.94,73.45 0 top
U28  ACS722LLCTR-05AB-T  [SOIC-8]  125.01,53.56 90 top
U29  ACS722LLCTR-05AB-T  [SOIC-8]  117.04,53.56 90 top
U30  ACS722LLCTR-05AB-T  [SOIC-8]  109.43,53.56 90 top
U31  MCP1700T-1802E/TT  [SOT95P237X112-3N]  23.35,53.9 0 top
U32  ACS722LLCTR-05AB-T  [SOIC-8]  101.83,53.56 90 top
U33  ACS722LLCTR-05AB-T  [SOIC-8]  48.52,47.26 90 top
U34  ACS722LLCTR-05AB-T  [SOIC-8]  28.14,47.26 90 top
U36  CPC1125N  [SOP-4]  19.04,91.18 0 top
U37  MC14541BDR2G  [SOIC14-3.9MM]  87.88,92.04 180 bottom
U38  CPC1017N  [SOP-4]  141.53,85.64 180 bottom
U39  CPC1017N  [SOP-4]  134.31,85.64 180 bottom
U40  MC14541BDR2G  [SOIC14-3.9MM]  99.97,91.23 180 bottom
U41  SIS413DN  [SIS413]  143.76,76.91 270 bottom
VRF  FIDUCIAL-1MM  [FD-1MM]  17.21,74.62 0 top
X2  1-2834019-3  [1-2834019-3]  126.84,37.38 90 top
X3  1-2834019-3  [1-2834019-3]  103.85,37.38 90 top
X4  1-2834019-3  [1-2834019-3]  80.87,37.38 90 top
X5  1-2834019-3  [1-2834019-3]  47.72,37.38 90 top
X6  1-2834019-3  [1-2834019-3]  24.71,37.38 90 top
X7  MICROSD  [MICROSD]  93.39,83.16 180 top
Y1  12MHz KX-7 20pF  [CRYSTAL-3.2-2.5]  53.7,77.62 270 top
Y2  32.768Khz  [RESONATOR_EPSON_FC_145]  40.61,86.81 0 top
Y3  32.768 kHz  [CRYSTAL-CITIZEN-CM2XXC]  99.44,94.79 90 top
Z1  CG0603MLC-05E  [CT/CN0603]  9.7,47.16 270 top
Z2  CG0603MLC-05E  [CT/CN0603]  11.73,47.16 270 top

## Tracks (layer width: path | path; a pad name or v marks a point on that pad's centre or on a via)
1D_INPUT
  Top 0.406: R122.1 92.89,61.53 92.34,62.08 91.84,62.08 C2.2 89.83,62.79 89.34,63.28 89.34,65.18 88.88,65.64 U20.2
1V8  (via drill 0.3 pad 0.61)
  Top 0.254: U22.2 55.94,36.94 C47.1 54.09,36.17 v53.77,36.49 53.89,36.37 53.89,31.8 56.24,29.45 56.24,28.43 52.56,24.75 52.56,20.18 54.96,17.77 54.96,14.32 54.53,13.89 54.53,7.54 54.91,7.16 57.96,7.16 58.49,7.69 JP2.1 | D1.3 24.02,48.08 25.19,46.91 29.76,46.91 32.81,43.86 v32.86,43.86 | v37.21,43.86 v40.69,43.86
  Top 0.406: C31.1 24.57,53.83 24.29,53.55 U31.2 24.29,51.32 D1.3
  Bottom 0.254: v32.86,43.86 v37.21,43.86 | v53.77,36.49 52.98,37.28 47.27,37.28 v40.69,43.86
  Bottom 0.406: JP2.1 61.51,9.32 63.81,9.32 JP3.1
3V  (via drill 0.3 pad 0.61)
  Top 0.2: v38.86,80.69 U1.52
  Top 0.254: RN1.5 RN1.6 RN1.7 RN1.8 24.26,99.4 22.44,97.58 22.44,95.91 23.69,94.66 JTAG.1 | 136.46,87.47 RN3.7 RN3.8 | 136.46,87.47 136.46,85.8 | C29.1 146.48,84.74 146.04,85.18 143.68,85.18 | 143.68,84.82 U11.5 143.68,85.18 | 136.46,85.8 143.22,85.8 143.68,85.34 143.68,85.18 | C9.1 C18.1 36.86,55.81 U1.125 | 130.21,66.48 130.21,65.48 | U1.105 24.93,60.84 C17.1 23.07,60.52 C6.+ | U1.57 36.36,77.16 v36.54,76.98 | C9.1 37.65,53.37 38.7,52.32 41.04,52.32 41.75,51.61 46.31,51.61 46.62,51.91 | C9.1 37.38,53.2 37.38,53.03 36.17,51.81 33.12,51.81 32.3,52.62 v32.3,53.13 | U1.11 49.55,64.34 50.22,63.66 51.72,63.66 52.62,62.76 C7.1 v53.67,62.75 C12.1 | L2.1 44.42,84.59 v44.42,85.58 | U1.62 33.86,77.52 v34.16,77.22 | U1.52 38.86,77.07 v39.15,76.78 | 136.46,85.8 136.46,85.77 | v138.17,87.27 136.67,87.27 136.46,87.47
  Top 0.3: v21.97,55.04 21,55.04 20.62,55.42 20.62,58.47 21.25,59.1 21.66,59.1 21.91,59.36 | C67.2 46.64,54.57 47.65,55.57 47.65,57.81 46.22,59.23 v46.22,62.38
  Top 0.305: v38.86,80.69 39.11,80.94 R10.1 39.11,82.9 38.75,83.26 C16.1 | v44.42,85.58 44.42,86.99 45.11,87.68 45.11,95.51 v45.04,95.78 | R80.2 57.41,94.67 59.53,92.55 61.97,92.55 62,92.58 v62.02,92.58
  Top 0.406: R80.2 ERASE.2 ERASE.1 C41.1 45.65,96.49 v45.04,95.78 | C11.1 R20.2 100.1,80.29 U2.8 100.1,85.41 99.46,86.05 84.61,86.05 v83.92,85.36 | U15.9 130.01,65.49 | 130.01,65.49 U15.6 | U15.10 130.49,66.76 130.21,66.48 130.21,65.69 130.01,65.49 | R12.2 R1.2 16.93,73.2 14.24,73.2 | 13.91,71.52 C44.1 14.4,71.03 U4.8 v14.4,65.68 | 13.91,71.52 13.91,71.62 | 17.29,79.53 15.09,79.53 14.24,78.68 14.24,73.2 | 17.29,79.53 JR1.2 | U17.6 115.85,65.62 117.12,66.89 U17.10 | v21.65,79.3 17.52,79.3 17.29,79.53 | R16.1 13.64,14.58 13.64,7.08 14.24,6.48 v17.04,6.48 | 18.54,6.48 18.74,6.68 18.74,7.43 J8.6 | U34.8 26.23,50.07 C68.2 27.27,51.78 v27.61,52.12 | v20.72,58.66 21.91,59.36 C6.+ | 76.78,78.33 C52.1 77.06,78.6 C51.+ 77.29,80.56 IC1.1 80.78,82.21 v83.92,85.36 | v82.92,86.82 87.69,91.6 X7.4 | v83.94,85.36 v83.92,85.36 | v42.74,95.88 42.7,95.88 41.2,97.38 32.46,97.38 30.37,95.29 30.37,94.38 29.05,93.06 24.66,93.06 23.79,93.92 JTAG.1 | 14.24,73.2 14.24,71.85 13.91,71.52
  Top 0.5: C63.2 U28.8 123.11,55.16 122.6,54.66 v122.09,54.66 115.36,54.66 | C67.2 46.62,53.57 46.62,51.91 U33.8 46.62,47.58 48.03,46.17 v50.47,46.17 | C66.2 99.93,59.67 U32.8 99.93,55.1 100.38,54.66 107.87,54.66 | C65.2 107.51,56.38 | 107.51,56.38 U30.8 | C64.2 115.13,56.37 U29.8 | U17.6 111.74,65.62 C55.1 | C55.1 C56.1 | U15.6 125.2,65.49 C53.1 C54.1 | JTAG.1 21.64,92.51 v21.64,88.48 | v21.65,79.3 L1.1 | 107.87,54.66 115.36,54.66 | C64.2 115.13,54.89 115.36,54.66 | 107.51,56.38 107.51,55.02 107.87,54.66 | v73.07,7.16 74.07,7.16 J6.6 | J9.6 117.59,7.48 v117.01,6.9 | J5.6 95.62,7.48 v95.04,6.9 | C64.2 112.08,59.72 v111.81,59.99 | v111.42,63.67 111.55,63.8 C55.1
  Top 0.508: 120.8,73.86 121,73.66 121,66.95 | 120.8,73.86 119.98,74.67 117.14,74.67 114.91,76.91 101.16,76.91 C11.1 | C54.1 122.09,65.86 121,66.95 | U17.10 120.94,66.89 121,66.95 | 136.46,85.77 134.31,83.61 134.31,80.46 | 120.8,73.86 130.96,73.86 134.31,77.21 134.31,78.33 | 134.31,80.46 134.31,78.33 | SJ3.1 133.9,80.87 134.31,80.46 | SJ3.3 131.77,78.63 132.18,78.23 v134.21,78.23 134.31,78.33
  Top 0.61: BR1.3 18.43,77.7 JR1.2 | J7.6 39.84,7.48 v39.44,7.08 | v17.04,6.48 18.54,6.48
  Bottom 0.254: v27.61,52.12 31.29,52.12 v32.3,53.13 | v46.22,62.38 46.6,62.75 v53.67,62.75 | v34.16,77.22 34.4,76.98 v36.54,76.98 36.74,76.78 v39.15,76.78 | U38.4 147.01,85.64 145.38,87.27 v138.17,87.27
  Bottom 0.305: v44.42,85.58 43.75,85.58 v38.86,80.69
  Bottom 0.406: v42.74,95.88 44.94,95.88 v45.04,95.78 | v27.61,52.12 24.68,55.04 v21.97,55.04 | v14.4,65.68 14.4,65.65 10.46,61.72 10.46,59.94 11.72,58.68 20.7,58.68 v20.72,58.66 | v83.94,85.36 82.92,86.38 v82.92,86.82 78.37,86.82 74.37,90.83 63.78,90.83 v62.02,92.58 | U41.8 U41.7 U41.6 U41.5 | v50.47,46.17 50.47,42.9 53.99,39.37 R59.1
  Bottom 0.5: v21.64,88.48 21.64,80.3 v21.65,79.3 | v39.44,7.08 57.4,7.08 58.34,6.14 72.06,6.14 v73.07,7.16 73.33,6.9 v95.04,6.9 v117.01,6.9 | v111.81,59.99 111.42,60.37 v111.42,63.67
  Bottom 0.508: U41.8 142.77,73.83 138.37,78.23 v134.21,78.23
  Bottom 0.61: v39.44,7.08 17.64,7.08 v17.04,6.48 | v117.01,6.9 129.33,6.9 138.35,15.92 138.35,47.8 131.49,54.66 v122.09,54.66
3V_U  (via drill 0.3 pad 0.61)
  Top 0.254: Q1.1 104.17,65.89 R95.2 104.2,64.66 103.43,63.9 96.82,63.9 96.51,64.21 R3.2 96.46,65.29 Q8.1 95.7,66.55 v95.5,66.75 | U21.2 65.46,40.4 65.22,40.64 64.41,40.64 63.9,40.13 63.86,40.13 C46.1 63.25,39.66 62.48,40.43 v62.17,40.43 | v54.25,45.41 54.25,46.66 C48.1 55.52,46.78 55.94,46.37 U22.19 | v10.46,72.44 10.58,72.55 R119.2 v9.14,73.86 | Q4.1 10.32,66 11.27,66.95 12.9,66.95 13.3,66.54 13.3,56.28 v13.41,56.18 | v37.99,44.9 39.72,44.9 v40.94,46.12 | v59.53,50.19 59.53,50.98 58.85,51.67 58.85,69.77 63.73,74.66 64.09,74.66 65.93,76.5 75.59,76.5 v76.09,75.99
  Top 0.3: Q1.1 104.17,64.58 104.19,64.56 106.73,64.56 107.11,64.94 107.11,70.28 110.28,73.45 v118.92,73.45
  Top 0.305: Q4.1 10.37,65.9 R117.2 | R119.2 10.63,73.91 Q5.1 | v121.33,76.12 125.29,76.12 134.86,85.69 RN3.5
  Top 0.406: U16.3 U16.2 | R62.2 80.39,78.81 U24.5 U24.6 81.72,77.55 C50.1 80.71,75.95 v80.16,76.5 | Q4.1 9.26,65.95 v9.24,65.93 | U31.3 23.35,54.55 22.96,54.15 21.33,54.15 v21.05,53.87 C42.1
  Top 0.61: U16.2 U16.1 SJ1.2 120.46,77.14 120.59,77.01
  Top 1.016: v121.33,76.12 121.33,77.14 U16.2
  Top 1.422: 143.04,49.08 143.58,49.08 PC3.+ D4.C
  Top 1.778: U5.4 v140.63,49.07 U5.2 143.03,49.07 143.04,49.08
  Bottom 0.254: R26.2 11.41,69.95 Q2.1 10.51,72.33 10.46,72.33 v10.46,72.44 | Q3.1 10.85,76.97 R115.2 9.23,73.86 v9.14,73.86 | v62.17,40.43 61.16,41.45 56.18,41.45 54.25,43.38 v54.25,45.41 52.52,47.14 41.96,47.14 v40.94,46.12 | v13.41,56.18 18.79,56.18 21.13,53.84 21.08,53.84 v21.05,53.87 30.02,44.9 v37.99,44.9 | v80.16,76.5 79.65,75.99 v76.09,75.99
  Bottom 0.3: v121.33,76.12 121.33,75.86
  Bottom 0.305: 52.52,47.14 54.35,48.97 58.42,48.97 59.53,50.08 v59.53,50.19
  Bottom 0.406: R26.2 11.36,68.05 v9.24,65.93 | v95.5,66.75 97.12,66.75 98.04,67.66 98.04,71.83 99.97,73.76 99.97,76.4 99.46,76.91 96.31,76.91 94.69,75.28 81.38,75.28 v80.16,76.5
  Bottom 1: v118.92,73.45 121.33,75.86
  Bottom 1.016: v121.33,76.12 136.32,76.12 139.24,73.2 139.24,50.47 v140.63,49.07
3V_U1  (via drill 0.3 pad 0.61)
  Top 0.508: SJ1.3 117.48,77.96 117.14,77.62 117.14,76.6 117.41,76.33 SJ1.1 | v133.29,79.75 132.99,80.06 SJ3.2 130.55,80.06 125.47,74.98 120.9,74.98 119.54,76.33 SJ1.1 | 118.88,76.32 SJ1.1
  Top 0.61: U16.5 U16.6 U16.7 U16.8 120.68,78.72 119.92,77.96 SJ1.3
  Bottom 0.406: U41.3 U41.2 U41.1 141.63,76.91 138.78,79.75 v133.29,79.75
5V  (via drill 0.3 pad 0.61)
  Top 0.254: R36.2 73.15,63.99 72.89,64.25 U18.14 | U19.14 62.33,64.25 R52.2 61.89,62 R48.1 | 12.54,83.48 12.64,83.48 14.54,85.38 | U21.19 65.46,44 65.2,43.73 63.61,43.73 C45.1 63.05,44.56 64.23,45.74 v64.23,46.66 | R86.1 30.31,91.03 32.61,91.03 32.75,90.89 U12.8 34.47,90.03 34.78,90.35 | SWS003.6 99.7,68.57 R57.2 | R57.2 99.7,69.56 | 99.7,71.29 R57.2 | v99.67,71.32 99.7,71.29 | R96.2 100.72,72.31 99.7,71.29 | 34.78,90.35 R66.1 | 34.78,90.35 R65.1 | U25.9 65.45,84.75 v64.77,84.07
  Top 0.305: v12.7,70.91 12.7,72.03 13.41,72.74 13.41,78.82 R120.2
  Top 0.406: U23.6 89.21,80.95 C49.1 | U23.6 U23.5 | U23.6 R61.2 R63.1 | U25.14 65.06,91.1 64.84,90.88 v64.84,89.91 64.84,89.78 | 64.84,89.78 64.84,88.88 65.16,88.56 U25.12 | U25.13 66.07,89.78 64.84,89.78 | 14.44,85.38 12.54,83.48 8.24,83.48 v7.94,83.18 SWS001.6 7.21,81.78 5.92,80.5 | 4.91,80.48 J11.1 5.92,80.5 | U20.14 82.16,64.37 R18.2 82.16,61.48 v82.15,60.77 | R33.1 78.42,62.45 v78.42,60.89 | R36.2 73.15,61.37 v72.66,60.88 | R2.1 131.87,87.8 126.03,81.96 | 126.03,81.96 v107.39,81.96 106.34,81.96 103.22,78.84 v103.22,77.82 | R48.1 61.97,61.97 61.56,61.57 59.74,61.57 59.43,61.26 59.43,51.91 64.23,47.11 v64.23,46.66 | 16.05,85.38 14.54,85.38 | 16.05,85.38 29.67,85.38 v29.88,85.18 | v61.77,84.22 61.75,84.25 61.84,84.28 61.95,84.39 61.95,85.58 | R118.2 12.8,70.81 v12.7,70.91 | v6.5,79.95 5.96,80.5 5.92,80.5 | R4.2 96.29,70.99 97.02,71.72 99.26,71.72 v99.67,71.32 | v93.16,68.17 93.15,68.16 R23.1 | R120.2 16.05,82.31 v16.05,84.12 16.05,85.38 | v141.63,72.84 144.35,70.12 D6.C | v126.03,78.99 v126.03,79 126.03,81.96 | v52.62,91.13 52.57,91.18 v46.76,91.18 | v31.29,91.23 31.09,91.03 30.31,91.03 | v61.87,89.91 61.95,89.83 61.95,85.58 | R27.2 91.48,64.94 v92.45,64.94 93.24,64.15 R122.2 | R19.2 86.58,74.4 U26.1 U26.6 | U25.5 61.95,86.02 61.95,85.58
  Top 0.5: R34.1 R35.2 | 65.84,75.06 R49.1 63.99,74.03 60.24,70.28 60.24,67.74 | 60.24,67.74 60.24,64.31 v60.37,64.18 60.75,63.8 R52.2 | R50.2 60.49,67.49 60.24,67.74 | R63.1 94.19,79.76 94.53,79.42 94.53,74.66 94.28,74.4 94.73,74.4 95.3,73.83
  Top 0.508: 95.3,73.83 95.3,71.58 R4.2 | 65.84,75.06 65.84,75.08 v66.34,75.59 72.94,75.59 73.31,75.22 R35.2 | 94.28,74.4 U26.6
  Top 1.016: L6.1 144.32,57.99 PC1.+ 144.35,64.74 D6.C
  Bottom 0.254: SWS002.6 12.05,82.46 12.53,82.94 R110.2 | R103.2 8.56,83.83 SWS001.6 7.22,82.46 v7.94,83.18 | J1.5 91.32,69.05 R121.2 | R60.1 64.76,46.66 v64.23,46.66
  Bottom 0.305: U37.14 91.13,85.75 92.65,84.22 103.02,84.22 103.22,84.42 | 103.22,84.42 103.42,84.63 107.28,84.63 107.59,84.32 107.59,82.09 107.39,81.88 v107.39,81.96 | U40.14 103.22,84.42
  Bottom 0.406: v64.84,89.91 v61.87,89.91 60.65,91.13 v52.62,91.13 | v61.77,84.22 64.61,84.22 v64.77,84.07 66.44,82.39 68.17,82.39 68.47,82.09 68.47,80.16 66.34,78.02 v66.34,75.59 | 78.54,60.77 v82.15,60.77 86.47,60.77 89.01,63.31 | 78.54,60.77 v78.42,60.89 78.41,60.88 | v60.37,64.18 61.18,64.18 64.48,60.88 v72.66,60.88 72.77,60.77 78.54,60.77 | U37.14 U37.13 U37.12 89.96,90.77 89.71,91.03 89.71,93.58 | U40.14 U40.13 U40.12 104.69,89.96 105.05,90.32 105.05,93.37 104.64,93.77 U40.9 99.53,93.77 98.26,92.5 U40.5 | U37.9 90.11,94.58 89.71,94.18 89.71,93.58 | R114.2 13,71.22 v12.7,70.91 | R116.2 6.6,79.84 v6.5,79.95 | v103.22,77.82 103.22,72.44 102.1,71.32 v99.67,71.32 99.67,66.64 97.96,64.94 92.94,64.94 | R121.2 92.27,69.06 v93.16,68.17 93.16,65.17 92.94,64.94 | R110.2 v16.05,84.12 | v141.63,72.84 137.16,77.31 127.7,77.31 v126.03,78.99 | v29.88,85.18 29.88,89.72 31.34,91.18 | 31.34,91.18 v46.76,91.18 | 31.34,91.18 v31.29,91.23 | 89.01,63.31 90.65,64.94 v92.45,64.94 92.94,64.94 | R22.1 89.01,63.41 89.01,63.31 | U37.5 89.44,93.31 89.71,93.58
5V_IN_ADC  (via drill 0.3 pad 0.61)
  Top 0.2: U1.91 28.27,67.84 v29.76,66.34 | v34.08,66.34 34.08,64.44 v36.11,62.4
  Top 0.406: R77.1 36.12,48.26 R78.2 33.77,48.74 v33.09,48.74
  Bottom 0.2: v29.76,66.34 v34.08,66.34
  Bottom 0.254: v36.11,62.4 36.11,58.01 33.7,55.6 33.7,49.35 v33.09,48.74
AREF
  Top 0.254: BR1.1 17.22,74.62 VRF.1
AVREF
  Top 0.254: U1.75 22.69,75.84 L3.2
  Top 0.406: L3.2 22.61,77.58 C19.1
AVREFL
  Top 0.61: L3.1 BR1.2 17.31,75.92 JR1.1 15.54,75.91 C40.1
BAT  (via drill 0.3 pad 0.61)
  Top 0.813: D3.A 107.08,93.64 v107.34,93.9
  Bottom 0.254: B2.POS2 130.22,90.32 130.22,90.22
  Bottom 1.016: B2.POS2 130.2,91.89 127.91,94.18 107.62,94.18 v107.34,93.9 | v107.34,93.9 107.31,93.9 107.28,93.87 107.32,93.87 v107.34,93.9
  Bottom 1.27: v107.34,93.9 B2.POS1
BOOTPULSE
  Top 0.254: U26.5 94.08,73.45 94.59,72.94 94.59,67.86 93.05,66.32 R27.1
  Top 0.406: U20.3 88.93,66.91 89.52,66.32 R27.1
BRD_RST
  Top 0.406: U23.3 86.51,76.91 86.94,76.48 92.54,76.48 93.01,76.95 R63.2
CONSOLE_RX  (via drill 0.3 pad 0.61)
  Top 0.2: U1.27 44.6,72.34 41.35,75.59 v41.35,76.8
  Top 0.254: J11.4 13.06,85 14.04,85.98 34.23,85.98 35.08,85.13 v35.04,85.13
  Bottom 0.2: v41.35,76.8 41.35,78.33 40.94,78.73 35.15,78.73
  Bottom 0.203: 35.15,78.73 34.23,79.65 34.23,84.32 v35.04,85.13
CONSOLE_TX  (via drill 0.3 pad 0.61)
  Top 0.2: v27.73,78.84 28.24,78.33 28.24,76.6 36.88,67.97 40.64,67.97 41.35,67.25 41.35,63.39 v40.33,62.38 | v14.22,82 14.21,81.99 9.65,81.99 9.66,82 J11.2 | U1.2 v47.09,59.84
  Bottom 0.2: 21.03,78.33 17.36,82 v14.22,82 | v47.09,59.84 42.87,59.84 v40.33,62.38
  Bottom 0.203: 21.03,78.33 21.38,77.98 26.88,77.98 v27.73,78.84
CS1
  Top 0.254: C58.2 116.04,58.52 116.04,60.8 117.33,62.08 134.01,62.08 134.81,62.88 134.81,69.28 133.52,70.57 U15.13
  Top 0.406: U29.7 C58.2
CS2  (via drill 0.3 pad 0.61)
  Top 0.254: C59.2 108.8,59.64 110.64,61.48 v115.21,61.48 | U15.3 125.56,69.3 v125.54,69.28
  Top 0.5: U30.7 C59.2
  Bottom 0.254: v115.21,61.48 121.81,61.48 122.6,62.28 122.6,66.34 v125.54,69.28
CS3
  Top 0.254: U15.11 133.56,68.03 134.01,67.58 134.01,63.08 133.61,62.68 110.05,62.68 108.5,61.13 101.27,61.13 100.88,60.75 100.88,58.58 C60.2
  Top 0.5: U32.7 101.2,58.14 C60.2
CS4  (via drill 0.3 pad 0.61)
  Top 0.254: C61.2 47.54,52.35 47.54,54.48 50.72,57.66 v50.72,58.34 | U17.1 110.8,71.97 108.39,69.56 108.39,63.31 107.36,62.4 99.23,62.4 98.34,61.51 98.34,56.89 93.7,52.24 70.91,52.24 v65.12,58.24
  Top 0.5: U33.7 47.89,51.96 C61.2
  Bottom 0.254: v50.72,58.34 50.97,58.09 64.56,58.09 v65.12,58.24
CS5  (via drill 0.3 pad 0.61)
  Top 0.254: U17.13 117.6,70.7 115.47,72.83 110.66,72.83 107.79,69.96 107.79,63.85 106.98,63.04 98.6,63.04 97.71,62.15 97.71,56.97 93.62,52.88 71.67,52.88 65.32,59.23 64.05,59.23 v63.8,58.97 | U34.7 27.51,48.78 27.73,48.56 v30.78,48.56 C62.2
  Bottom 0.254: v63.8,58.97 63.47,58.64 51.94,58.64 51.23,59.36 49.37,59.36 48.1,58.09 42.84,58.09 34.74,49.98 34.74,48.26 34.03,47.54 31.8,47.54 v30.78,48.56
CS_5V
  Top 0.254: U15.1 128.77,71.84 130.01,73.08 134.31,73.08 135.51,71.88 135.51,62.18 134.71,61.38 124.64,61.38 124,60.74 124,58.57 C57.2
  Top 0.406: U28.7 C57.2
CS_FET_CTRL  (via drill 0.3 pad 0.61)
  Top 0.254: U18.8 74.86,71.87 75.53,72.54 v75.53,72.71 | v93.01,54.02 93.01,55.93 85.14,63.8 85.14,68.25 v85.52,68.63 | R9.1 79.53,17.97 v78.79,18.71 | v87.17,43.66 87.17,35.05 79.09,26.97 v79.09,23.44
  Bottom 0.254: v93.01,54.02 87.17,48.18 v87.17,43.66 | v79.09,23.44 78.79,23.13 v78.79,18.71 | v75.53,72.71 75.74,72.51 82.31,72.51 84.24,70.58 84.24,69.9 v85.52,68.63
CS_LAT_CLK  (via drill 0.3 pad 0.61)
  Top 0.2: U18.11 71.28,68.06 v71.26,68.08 | U1.63 33.36,76.84 39.91,70.29 v39.91,70.04
  Bottom 0.2: v71.26,68.08 68.93,70.4 63.42,70.4 62.1,69.08 40.87,69.08 v39.91,70.04
  Bottom 0.203: R56.2 79.3,68.08 v71.26,68.08
CS_LAT_D  (via drill 0.3 pad 0.61)
  Top 0.2: U18.12 v71.27,66.79 v71.26,66.78 | U1.64 32.86,76.58 38.71,70.73 v38.71,70.07
  Bottom 0.2: v71.26,66.78 68.14,69.9 63.8,69.9 62.58,68.68 40.03,68.68 38.71,69.99 v38.71,70.07
CS_RELAY_CTRL
  Top 0.2: U18.9 73.44,70.6 74.26,69.78 74.26,58.62 75.08,57.81 | U10.4 86.52,56.32 85.39,57.45 80.16,57.45 79.9,57.45
  Top 0.203: 75.08,57.81 75.43,57.45 80.16,57.45
CS_RELAY_RETURN  (via drill 0.3 pad 0.61)
  Top 0.254: U10.15 86.52,44.25 86.15,43.89 86.15,35.25 77.97,27.07 v77.97,23.44
  Bottom 0.254: K3.1 76.14,16.3 77.97,18.13 v77.97,23.44
D+  (via drill 0.3 pad 0.61)
  Top 0.2: R7.2 50.34,80.17 50.34,79.98 49.77,79.41 47.61,79.41 v47.09,78.89 U1.37 | RN2.1 13.07,50.15 14.78,51.86 14.78,62.02 v15.29,62.53
  Bottom 0.2: v15.29,62.53 23.79,71.04 23.79,73.98 24.28,74.47 | v47.09,78.89 47.09,76.81 45,74.72 32.05,74.72
  Bottom 0.203: 32.05,74.72 24.53,74.72 24.28,74.47
D-  (via drill 0.3 pad 0.61)
  Top 0.2: 46.4,77.88 47.39,77.88 47.89,78.38 R6.2 | 46.4,77.88 46.04,77.88 45.86,78.06 U1.38 | RN2.2 13.11,50.95 14.27,52.12 14.27,62.23 v14.09,62.4 | v46.27,77.59 46.27,77.75 46.4,77.88
  Bottom 0.2: v46.27,77.59 46.27,77.26 44.19,75.18 31.69,75.18 | 23.97,74.87 23.03,73.94 23.03,71.55
  Bottom 0.203: 23.03,71.55 23.03,71.09 22.45,70.51 14.63,62.89 14.14,62.4 v14.09,62.4 | 31.69,75.18 24.28,75.18 23.97,74.87
D_N
  Top 0.2: RN2.7 10.7,50.95 11.04,50.61 11.04,48.88 11.73,48.19 Z2.1
  Top 0.254: J3.2 10.33,50.86 RN2.7
D_P
  Top 0.254: J3.3 10.36,50.21 RN2.8 10.42,48.89 Z1.1
EE_RST  (via drill 0.3 pad 0.61)
  Top 0.2: U1.19 56.53,68.34 64.56,76.37 v64.69,76.37 | v62.78,78.28 62.78,91.42 63.24,91.88 63.24,98.69
  Top 0.406: EERST.2 63.24,98.69 EERST.1 R80.1
  Bottom 0.2: v64.69,76.37 v62.78,78.28
EP_BOOT_SEL  (via drill 0.3 pad 0.61)
  Top 0.2: U1.98 25.54,64.34 v24.48,65.4 | v20.11,60.37 19.86,60.12 19.86,50.54 23.29,47.11 R32.2
  Bottom 0.2: v20.11,60.37 20.11,63.04 22.47,65.4 v24.48,65.4
EP_FET_CTRL  (via drill 0.3 pad 0.61)
  Top 0.2: 80.56,68.98 80.56,58.98 v80.82,58.72
  Top 0.203: U18.6 78.98,70.6 80.56,69.02 80.56,68.98
  Top 0.254: v94.53,55.67 v88.95,61.26 | R64.1 101.43,19.1 90.98,19.1 89.58,20.49 89.58,22.27 92.5,25.19 98.98,25.19 100.78,26.99 100.78,44.7 104.82,48.74 104.82,52.14 104.47,52.5 96.84,52.5 v96.08,51.73
  Bottom 0.254: v88.95,61.26 86.41,58.72 v80.82,58.72 | v94.53,55.67 96.08,54.12 v96.08,51.73
EP_LAT_CLK  (via drill 0.3 pad 0.61)
  Top 0.2: U18.3 76.47,66.79 | U1.60 34.86,76.48 41.08,70.27 v41.09,70.27
  Top 0.203: 76.47,66.79 75.24,68.01 v75.24,70.54
  Bottom 0.2: v41.09,70.27 41.86,69.49 61.62,69.49 63.04,70.91 72.84,70.91
  Bottom 0.203: 72.84,70.91 74.87,70.91 v75.24,70.54 75.78,70 R98.1
EP_LAT_D  (via drill 0.3 pad 0.61)
  Top 0.2: U1.116 32.36,58.65 v32.56,58.85 | U18.2 77.01,65.52 v76.56,65.07
  Bottom 0.2: v32.56,58.85 34.21,58.85 35.35,59.99 35.35,62.91 38.78,66.34 63.8,66.34 63.81,66.33 63.82,66.33 | v76.56,65.07 76.5,65.01 76.5,64.31 75.79,63.6 66.55,63.6 63.82,66.33 | 63.82,66.33 63.8,66.33
EP_RELAY_CTRL
  Top 0.2: U18.5 79.61,69.33 80.06,68.88 80.06,58.34 80.06,58.21 80.31,57.96 86.28,57.96 87.79,56.45 U10.3
EP_RELAY_RETURN  (via drill 0.3 pad 0.61)
  Top 0.254: K2.1 92.76,16.3 88.95,20.11 88.95,22.65 92.25,25.95 98.47,25.95 99.77,27.25 99.77,29.36 96.31,32.81 v96.31,39.29 | v93.14,45.64 91.11,47.67 87.93,47.67 87.79,47.53 U10.16
  Bottom 0.254: v96.31,39.29 96.31,42.46 v93.14,45.64
ERASE_S  (via drill 0.3 pad 0.61)
  Top 0.2: U1.130 39.38,57.3 v39.38,58.52 | v39.11,62.48 40.74,64.11 40.74,66.75 40.13,67.36 36.67,67.36 27.83,76.19 27.83,77.52 26.82,78.53 26.82,83 v27.43,83.61
  Top 0.254: J11.6 11.29,88 12.21,87.08 25.07,87.08 v25.23,87.23 25.33,87.13 35.62,87.13 36.27,87.78 36.27,90.32 37.59,91.64 39.62,91.64 40.33,92.35 40.33,94.68 v40.3,94.71 | v55.47,97.43 55.47,94.2 ERASE.3 | ERASE.4 46.78,94.89 v45.94,94.89
  Top 0.406: ERASE.3 ERASE.4
  Bottom 0.2: v39.11,62.48 39.11,58.78 v39.38,58.52 | v27.43,83.61 27.43,85.07
  Bottom 0.203: 27.43,85.07 27.39,85.07 v25.23,87.23
  Bottom 0.254: U38.3 147.33,95.79 144.67,98.45 136.44,98.45 134.82,96.82 109.42,96.82 106.99,99.26 79.45,99.26 78.96,99.74 57.48,99.74 55.47,97.73 v55.47,97.43 | v45.94,94.89 45.76,94.71 v40.3,94.71
GND  (via drill 0.3 pad 0.61)
  Top 0.2: U1.106 27.72,60.34 28.04,60.65 v28.04,60.96 | IC1.11 70.07,88.56 69.59,88.08 69.59,85.03 69.87,84.75 IC1.14 | 83.51,72.64 83.21,72.64 82.9,72.94 82.9,75.08 83.62,75.79 C50.2
  Top 0.203: 83.51,72.64 83.94,72.64 v84.21,72.37
  Top 0.254: SWS003.4 102.07,67.42 v102.41,67.76 | C12.2 C7.2 C34.2 50.79,64.84 U1.12 47.14,64.84 v46.92,65.06 | C9.2 C18.2 39.21,55.25 39.21,55.57 38.6,56.18 37.59,56.18 37.36,56.41 U1.126 37.36,58.49 v37.69,58.82 | C32.2 C27.2 | U1.33 50.23,75.34 51,74.57 51,71.52 51.43,71.09 C39.- | Y1.2 52.78,76.24 53.64,75.38 55.57,75.38 56.38,74.57 | 56.38,74.57 56.38,72.13 55.91,71.65 C38.2 | C21.1 57.64,76.23 57.2,75.79 57.2,75.38 56.38,74.57 | Y1.4 54.63,77.95 54.96,77.62 57.68,77.62 | 37.42,84.59 R5.2 | JTAG.9 28.88,94.1 28.44,93.67 26.61,93.67 26.31,93.97 26.31,94.64 JTAG.5 | C37.- 46.91,85.33 45.07,83.48 43.35,83.48 C35.2 42.31,83.87 41.86,83.41 U1.46 | U1.74 25.25,76.34 24.32,77.27 24.32,80.14 C26.2 23.7,81.34 22.86,82.19 22.86,82.55 C36.- | R85.2 R81.2 | X7.6 89.89,95.42 89.4,95.91 84.32,95.91 79.55,91.13 v78.84,91.13 77.31,91.13 IC1.8 | C47.2 55.16,32.61 56.89,30.88 56.89,28.14 53.44,24.68 v53.44,24.07 | U1.44 42.86,77.66 v43.37,77.14 | U1.58 35.86,79.75 35.35,80.26 v35.15,80.26 | U1.54 37.86,77.82 v38.09,77.58
  Top 0.305: v79.85,95.91 79.79,95.97 X7.MT2 | IC1.14 72.47,84.75 v73.22,84.01 | IC1.8 76.07,91.1 73.53,88.56 IC1.11 | C16.2 33.24,82.95 C28.2
  Top 0.406: U36.2 19.04,89.26 v18.89,89.5 | Z2.2 Z1.2 8.79,46.16 8.33,46.63 8.33,48.56 7.97,48.91 J3.5 J3.4 | EERST.4 v59.74,94.19 v59.74,94.18 | EERST.3 69.2,92.95 v69.29,92.86 | C21.1 57.68,76.51 57.68,77.62 C22.2 57.68,80.18 | 57.68,80.18 56.51,81.35 C25.2 R8.2 53.67,83.07 51.96,84.78 C20.2 | U25.7 v59.63,82.12 57.68,80.18 | C39.- 54.57,71.09 C38.2 | 67.57,84.75 R28.2 | R58.1 64.08,81.86 | C51.- 74.76,79.88 C52.2 | U18.7 78.98,71.87 79.45,72.33 v79.45,73.25 | U24.2 U23.2 87.65,78.81 87.78,78.94 87.78,80.16 86.91,81.03 C49.2 | U26.2 88.79,73.45 87.83,72.49 U20.7 | U26.4 93.24,71.09 R25.2 | 143.68,80.77 145.99,80.77 146.48,81.25 C29.2 | U11.2 143.68,80.77 | 143.68,80.77 138.78,80.77 v138.17,81.38 | C24.2 C23.2 38.12,90.25 37.69,89.81 37.69,85.34 37.42,85.08 R5.2 | C36.- 20.07,82.94 v20.01,83 | C33.2 22.5,65.51 C8.- | C6.- 23.87,56.74 C31.2 | X7.6 89.89,91.96 92.75,89.11 92.96,89.11 | 92.96,89.11 U2.4 | 92.96,89.11 92.99,89.14 X7.MT1 93.7,95.99 C15.2 96.9,97.54 Y3.P$3 Y3.P$2 102.01,97.54 C14.2 106.15,98.59 L13.C | C37.- 46.16,85.53 v45.3,86.39 | R82.2 65.61,13.54 R87.1 68.03,11.84 R97.1 69.44,11.93 v69.49,11.98
  Top 0.61: C37.- 48.48,85.53 C20.2 | 103.12,56.69 102.79,56.36 U32.6 U32.5 104.42,56.36 v104.75,56.69 v105.66,56.69 105.71,56.73 C65.1 | 103.12,58.15 C60.1 103.06,58.56 C66.1 | U30.6 110.71,56.36 U30.5 | C59.1 110.71,58.16 | U29.6 118.26,56.36 U29.5 | 126.18,56.38 126.16,56.36 U28.6 126.39,56.36 U28.5
  Top 0.8: L11.C v124.45,98.59 L10.C L9.C L4.C L8.C L.C L7.C L12.C L13.C | ON.C ON1.C TX1.C 129.73,98.65 v130.86,98.65 | 103.12,56.69 103.12,58.15 | 110.71,58.16 110.71,56.36
  Top 0.813: 118.26,56.36 118.26,58.11 C58.1 118.21,58.43 C64.1 117.56,60.35 v119.68,60.35 v120.7,60.35 | 110.71,58.16 110.97,58.41 v112.06,58.41 v112.97,58.41 | C63.1 126.1,59.86 v126.18,59.94 126.18,58.21 C57.1 126.18,58.2 126.18,56.38
  Top 1: R68.1 119.42,33.57 121.84,35.99 X2.2 | R75.1 40.42,34.62 X5.2
  Top 1.016: D4.A 141.51,56.08 135.12,56.08 132.37,58.83 PC2.-
  Top 1.27: PC2.- 128.86,58.83 126.39,56.36 | D4.A 145.34,53.99 146.3,53.03 146.3,46.95 PC3.- 141.1,46.76 U5.1 | J9.4 123.59,9.49 | 123.59,9.49 v124.05,9.95 | J5.4 v101.49,9.95 v100.58,9.95 | J6.4 79.39,8.89 v79.04,9.24 v79.85,9.24 | J7.4 45.79,9.52 v46.22,9.95 v45.31,9.95 | J8.4 23.69,9.26 v24.18,9.75 v23.26,9.75 | 123.59,9.49 123.59,9.5 v123.13,9.95
  Top 2.45: J10.P$2 146.34,41.52 PC3.- 144.31,43.55 PC5.-
  Bottom 0.203: R98.2 80.75,70.46 v80.75,70.65
  Bottom 0.254: v37.69,58.82 37.79,58.82 37.99,59.03 | v35.15,80.26 35.05,80.77
  Bottom 0.406: JTAG.5 JTAG.3 | 139.9,88.18 139.9,89.58 R106.2 139.47,90.01 R107.2 | U13.2 14.92,38.41 15.64,37.69 15.64,34.64 14.99,33.99 U14.2
  Bottom 0.508: R73.1 98.36,37.87 X3.2
  Bottom 0.8: v130.86,98.65 130.8,98.59 v124.45,98.59
  Bottom 2.45: X2.2 X3.2 X4.2 | X5.2 X6.2
  other vias: 32.71,54.66 123.64,72.94 119.78,72.74 72.43,79.58 87.85,79.74 50.89,84.76 37.68,85.78 39.31,55.98 24.99,66.95 30.95,49.79 23.26,58.21 32.77,46.03 89.29,72.47 80.16,48.76 65.73,50.19 78.84,11.68 79.95,11.68 64.82,37.49 86.05,48.86 61.36,47.43 54.96,50.08 75.08,61.97 49.37,38.5 49.47,21.53 46.32,17.06 50.38,48.41 4.26,84.73 15.84,78.74 19.6,78.33 15.64,66.44 20.92,72.64 31.9,95.4 67.87,83.35 64.4,72.98 104.74,76.03 116.93,64.34 65.21,61.74 41.65,45.31 8.43,49.17 13.1,52.52 35.76,94.99 33.41,80.8 70,49.68 72.54,57.4 77.62,59.74 96.41,63.09 110.84,86.05 23.06,53.01 30.7,92.8 44.16,91.94 108.86,40.36 138.06,7.26 132.16,23.76
  pour Bottom: 2.84,5.38 148.84,5.38 148.84,100.38 2.84,100.38
  pour Top: 2.84,5.38 148.84,5.38 148.84,100.38 2.84,100.38
INA1  (via drill 0.3 pad 0.61)
  Top 0.203: U12.1 32.75,95.33 33.52,96.11 36.47,96.11 v37.69,94.89 | v47.75,92.05 53.84,92.05 54.15,91.74 54.15,87.37 54.86,86.66 v58.31,86.66
  Top 0.254: v102.71,69.79 102.45,69.54 R57.1
  Top 0.3: R57.1 101.57,69.51 SWS003.5
  Bottom 0.203: v37.69,94.89 39.52,93.06 47.54,93.06 47.75,92.86 v47.75,92.05
  Bottom 0.254: v58.31,86.66 58.72,86.25 72.64,86.25 75.69,83.21 83.6,83.21 84.11,82.7 99.67,82.7 100.38,82.7 100.67,82.7 100.98,83 103.93,83 106.07,80.87 106.07,73.15 v102.71,69.79
INA2  (via drill 0.3 pad 0.61)
  Top 0.203: U12.3 31.75,93.62 31.49,93.87 30.78,93.87 29.38,92.48 23.79,92.48 23.06,91.74 23.06,88.29 22.55,87.78 13.61,87.78 v13.2,88.18
  Bottom 0.203: 10.66,84.12 10.66,85.64 v13.2,88.18
  Bottom 0.254: SWS002.5 10.66,84.12 R110.1
INA3  (via drill 0.3 pad 0.61)
  Top 0.203: U12.6 31.75,89.25 30.37,87.88 v29.05,87.88
  Bottom 0.203: R103.1 6.67,87.34 9.65,90.32 23.26,90.32 26.21,87.37 28.54,87.37 v29.05,87.88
